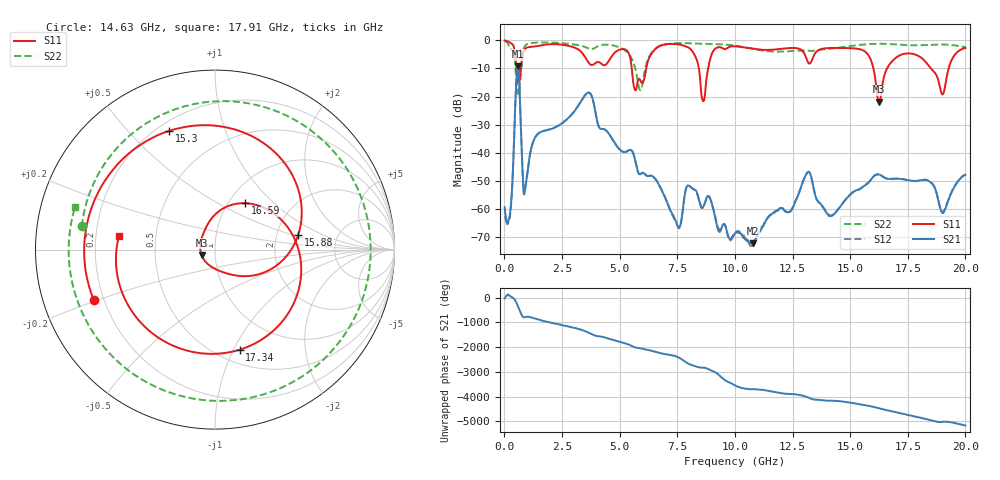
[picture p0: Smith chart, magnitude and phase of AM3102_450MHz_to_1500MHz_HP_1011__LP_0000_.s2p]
!Agilent Technologies,E8364B,MY43040894,A.07.50.67
!Agilent E8364B: A.07.50.67
!Date: Thursday, January 11, 2018 06:22:52
!Correction: S11(Full 2 Port(1,2))
!S21(Full 2 Port(1,2))
!S12(Full 2 Port(1,2))
!S22(Full 2 Port(1,2))
!S2P File: Measurements: S11, S21, S12, S22:
# Hz S  dB  R 50
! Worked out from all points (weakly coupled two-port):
!   1601 points, 10 MHz to 20 GHz, reference 50 ohm
!   highest |S21| = -9.20 dB at 597.2 MHz (marker M1); lowest = -72.2 dB at 10.78 GHz (marker M2)
!   lowest |S11| = -21.8 dB at 16.25 GHz (marker M3), VSWR 1.18, Z = 43 - j2.62 ohm
!   |S11| at or under -10 dB: 5.526 GHz to 6.156 GHz (629.5 MHz wide, 10.8 % of centre); 16.01 GHz to 16.6 GHz (592 MHz wide, 3.63 % of centre); 18.5 GHz to 19.27 GHz (767.5 MHz wide, 4.06 % of centre)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
!   |S22| runs from -19.2 to -0.3 dB; largest |S21 - S12| = 0.0012
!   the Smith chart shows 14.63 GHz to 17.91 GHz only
!   S11 on the Smith chart (normalised r, x): 14.63 GHz: 0.16, -0.19; 15.3 GHz: 0.25, +0.66; 15.88 GHz: 2.64, +0.54; 16.59 GHz: 1.19, +0.68; 17.34 GHz: 0.63, -1.06; 17.91 GHz: 0.30, +0.07
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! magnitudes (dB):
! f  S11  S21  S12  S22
! 10 MHz  -0.1  -59.3  -62.5  -0.3
! 259.9 MHz  -0.9  -60.5  -61.5  -2.9
! 597.2 MHz  -14.7  -9.2  -9.2  -18.9
! 897.1 MHz  -3.0  -52.9  -52.8  -1.9
! 3.346 GHz  -4.2  -21.4  -21.4  -2.0
! 5.895 GHz  -14.2  -47.6  -47.6  -17.8
! 6.682 GHz  -2.2  -51.0  -51.0  -2.4
! 8.106 GHz  -3.4  -52.3  -52.3  -1.1
! 8.618 GHz  -21.6  -59.3  -59.4  -1.2
! 10.01 GHz  -2.1  -68.6  -68.4  -1.9
! 10.78 GHz  -3.0  -72.2  -73.1  -3.0
! 13.34 GHz  -7.1  -49.5  -49.6  -3.8
! 14.63 GHz  -2.7  -58.5  -58.4  -2.5
! 15.3 GHz  -3.0  -53.3  -53.2  -1.7
! 15.88 GHz  -6.6  -49.8  -49.8  -1.3
! 16.25 GHz  -21.8  -47.7  -47.7  -1.2
! 16.59 GHz  -10.2  -49.2  -49.2  -1.3
! 16.68 GHz  -9.0  -49.3  -49.3  -1.3
! 17.34 GHz  -4.8  -49.5  -49.4  -1.6
! 17.91 GHz  -5.4  -50.0  -50.0  -1.8
! 19.01 GHz  -19.2  -61.3  -61.2  -1.5
! 20 GHz  -2.7  -47.9  -47.8  -2.4
